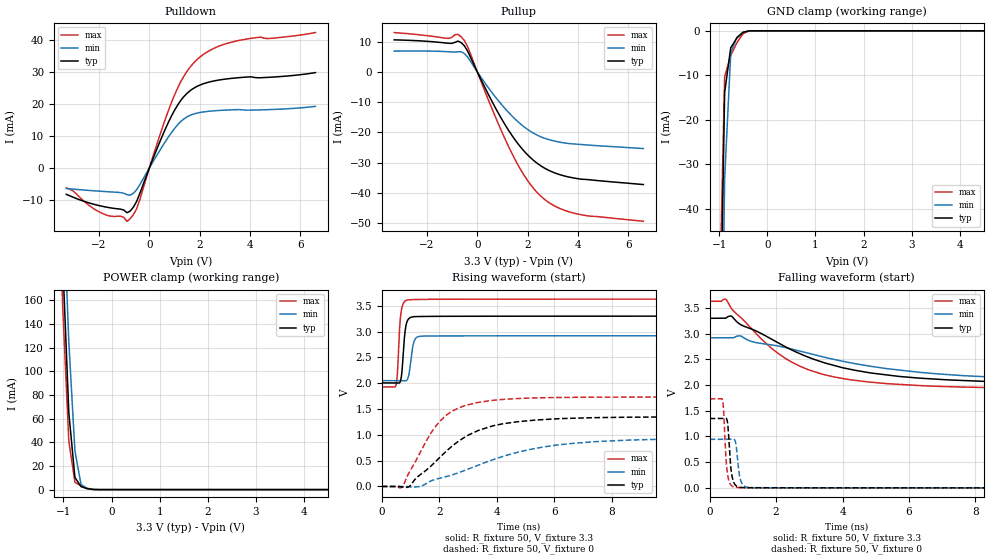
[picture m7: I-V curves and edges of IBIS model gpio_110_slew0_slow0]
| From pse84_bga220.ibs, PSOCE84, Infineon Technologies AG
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[Model] gpio_110_slew0_slow0
Model_type I/O
Enable   Active-High
Vinl  =  0.99
Vinh  =  2.31
Vmeas =  1.65
Cref  =  15e-12
| Capacitance   typ   min   max
C_comp   1.09946e-12   1.086232e-12   1.114407e-12
| Variables   typ   min   max
[GND Clamp Reference]   0   0   0
[POWER Clamp Reference]   3.3   2.92   3.63
[Pulldown Reference]   0   0   0
[Pullup Reference]   3.3   2.92   3.63
[Temperature Range]   25   125   -40
[Voltage Range]   3.3   2.92   3.63
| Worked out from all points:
|   slope of the pulldown table from 0 to 0.495 V, typ, clamps not added: 51.4 ohm
|   slope of the pullup table from 0 to 0.495 V, typ, clamps not added: 59.6 ohm
|   GND clamp passes 1 mA (typ) near -0.57 V on its own axis
|   POWER clamp passes 1 mA (typ) near -0.52 V on its own axis
|   falling waveform, R_fixture 50, V_fixture 3.3: 20-80 % time 3.15ns typ, 4.56ns min, 2.14ns max; typ from 3.3 V to 2.01 V
|   falling waveform, R_fixture 50, V_fixture 0: 20-80 % time 97ps typ, 106ps min, 91.3ps max; typ from 1.35 V to 0 V
|   rising waveform, R_fixture 50, V_fixture 3.3: 20-80 % time 111ps typ, 130ps min, 100ps max; typ from 2.01 V to 3.3 V
|   rising waveform, R_fixture 50, V_fixture 0: 20-80 % time 1.89ns typ, 3.29ns min, 1.22ns max; typ from 0 V to 1.35 V
[GND Clamp]
| Voltage   I(typ)   I(min)   I(max)
-1.65V    -892.5mA   -911.9mA   -883.9mA
-1.015V   -92.32mA   -129.7mA   -71.28mA
-888.3mV  -13.83mA   -33.21mA   -10.31mA
-761.4mV  -3.792mA   -4.944mA   -5.509mA
-634.5mV  -1.622mA   -1.436mA   -2.707mA
-507.6mV  -326.2uA   -352.3uA   -651.6uA
-380.7mV  -13.48uA   -32.14uA   -19.55uA
-253.8mV  -189.4nA   -1.276uA   -466.7nA
6.6V      0A         0A         0A
[POWER Clamp]
| Voltage   I(typ)   I(min)   I(max)
-1.523V   838.1mA    872.9mA    823.9mA
-1.142V   346.5mA    405.1mA    310.5mA
-1.015V   193mA      257.4mA    153.9mA
-888.3mV  64.97mA    124.9mA    40.96mA
-761.4mV  10.28mA    32.7mA     6.184mA
-634.5mV  2.553mA    4.346mA    3.067mA
-507.6mV  805.9uA    960.7uA    1.159mA
-253.8mV  1.454uA    10.02uA    1.678uA
6.6V      0A         0A         0A
[Pulldown]
| Voltage   I(typ)   I(min)   I(max)
-3.3V     -8.212mA   -6.392mA   -6.208mA
-2.03V    -11.66mA   -7.202mA   -13.53mA
-1.142V   -12.83mA   -7.672mA   -15.01mA
-888.3mV  -13.95mA   -8.321mA   -16.62mA
-507.6mV  -10.46mA   -6.8mA     -12.77mA
455.2mV   8.891mA    5.99mA     11.13mA
1.024V    18.33mA    12.55mA    23.2mA
1.366V    22.23mA    15.28mA    28.56mA
1.821V    25.16mA    16.99mA    33.26mA
2.503V    27.06mA    17.8mA     37.1mA
3.3V      28mA       18.16mA    39.33mA
6.6V      29.77mA    19.23mA    42.26mA
[Pullup]
| Voltage   I(typ)   I(min)   I(max)
-3.3V     10.56mA    6.84mA     12.97mA
-1.142V   9.434mA    6.628mA    11.05mA
-761.4mV  10.16mA    6.628mA    12.36mA
-634.5mV  9.61mA     6.615mA    11.54mA
-380.7mV  6.812mA    4.862mA    8.263mA
682.8mV   -11.29mA   -7.908mA   -14.14mA
1.479V    -22.2mA    -15.4mA    -28.59mA
2.048V    -27.81mA   -19.3mA    -36.47mA
2.731V    -32.06mA   -22.09mA   -42.48mA
3.3V      -34.01mA   -23.26mA   -45.19mA
4.051V    -35.35mA   -23.94mA   -47.06mA
6.6V      -37.22mA   -25.33mA   -49.35mA
[Ramp]
dV/dt_r   0.809557/1.8924n  0.566599/3.2914n  1.03932/1.22294n
dV/dt_f   0.776057/3.14843n  0.521389/4.55877n  1.02156/2.141n
R_load = 50
[Falling Waveform]
R_fixture = 50
V_fixture = 3.3
V_fixture_min = 2.92
V_fixture_max = 3.63
| Time   V(typ)   V(min)   V(max)
0s        3.3V       2.92V      3.63V
493.2ps   3.306V     2.92V      3.666V
654.3ps   3.343V     2.92V      3.492V
918.6ps   3.182V     2.958V     3.327V
2.019ns   2.835V     2.765V     2.637V
2.695ns   2.618V     2.665V     2.374V
3.71ns    2.389V     2.505V     2.163V
6.311ns   2.136V     2.249V     1.991V
12.77ns   2.021V     2.083V     1.929V
800ns     2.007V     2.051V     1.927V
[Falling Waveform]
R_fixture = 50
V_fixture = 0
V_fixture_min = 0
V_fixture_max = 0
| Time   V(typ)   V(min)   V(max)
0s        1.349V     944.3mV    1.732V
386.4ps   1.349V     944.2mV    1.713V
418.9ps   1.349V     944.2mV    1.525V
534.2ps   1.287V     944.3mV    286.5mV
632ps     427.3mV    944.3mV    61.99mV
775.8ps   52.28mV    897.4mV    10.29mV
899.4ps   11.65mV    238.5mV    4.503mV
1.01ns    4.225mV    50.15mV    3.877mV
1.792ns   2.137mV    1.535mV    1.819mV
800ns     14.69nV    476.2nV    8.32nV
[Rising Waveform]
R_fixture = 50
V_fixture = 3.3
V_fixture_min = 2.92
V_fixture_max = 3.63
| Time   V(typ)   V(min)   V(max)
0s        2.007V     2.051V     1.927V
496.5ps   2.007V     2.051V     1.965V
546.9ps   2.007V     2.051V     2.215V
646.7ps   2.035V     2.051V     3.256V
699.9ps   2.213V     2.051V     3.463V
764.2ps   2.714V     2.051V     3.562V
884.3ps   3.201V     2.067V     3.612V
1.166ns   3.291V     2.859V     3.622V
1.828ns   3.296V     2.916V     3.627V
800ns     3.3V       2.92V      3.63V
[Rising Waveform]
R_fixture = 50
V_fixture = 0
V_fixture_min = 0
V_fixture_max = 0
| Time   V(typ)   V(min)   V(max)
0s        14.93nV    475.9nV    8.654nV
714.1ps   -10.71mV   43.07uV    -10.75mV
954.9ps   -2.123mV   -5.591mV   272.5mV
1.749ns   415.6mV    115.7mV    1.068V
2.225ns   673.4mV    188.4mV    1.374V
2.676ns   879.3mV    267.9mV    1.523V
4.163ns   1.21V      574.1mV    1.685V
5.757ns   1.3V       776.9mV    1.721V
7.865ns   1.337V     879.5mV    1.731V
800ns     1.349V     944.3mV    1.732V
